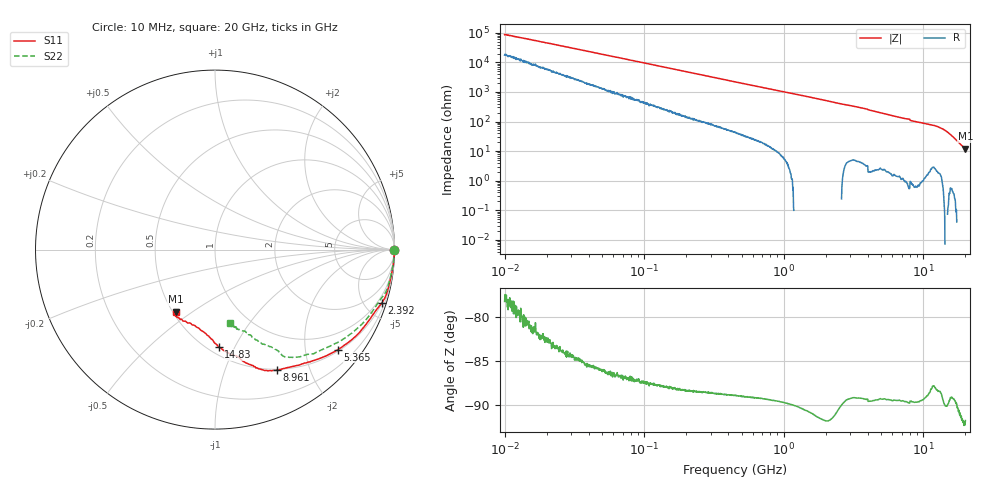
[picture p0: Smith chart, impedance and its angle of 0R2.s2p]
!Keysight Technologies,P5008B,MY61100088,A.16.20.02
!Date: Monday, October 30, 2023 15:49:30
!Correction: S11(C  2-Port  )
!S21(C  2-Port  )
!S12(C  2-Port  )
!S22(C  2-Port  )
!S2P File: Measurements: S11, S21, S12, S22:Log Frequency Sweep
# Hz S  dB  R 50
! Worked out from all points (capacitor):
!   1601 points, 10 MHz to 20 GHz, reference 50 ohm
!   read as one part in series: C = 181 fF near 10.39 MHz
!   lowest |Z| = 11.9 ohm at 20 GHz (marker M1)
!   S11 on the Smith chart (normalised r, x): 10 MHz: open; 2.392 GHz: 0.52, -6.36; 5.365 GHz: 0.54, -2.72; 8.961 GHz: 0.49, -1.52; 14.83 GHz: 0.56, -0.87; 20 GHz: 0.52, -0.43
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1e7  0.00 -0.1  -58.83 78.2  -58.91 78.9  -0.00 -0.1
3.555162e7  -0.00 -0.3  -48.41 84.8  -48.41 84.9  -0.00 -0.2
1.263918e8  -0.01 -1.0  -37.66 86.8  -37.66 86.9  -0.01 -0.8
4.472136e8  -0.02 -3.4  -26.88 85.7  -26.88 85.7  -0.02 -2.9
9.518201e8  -0.05 -7.1  -20.56 83.0  -20.57 83.0  -0.06 -6.1
1.589917e9  -0.09 -11.6  -16.38 80.1  -16.39 80.1  -0.10 -10.0
2.39224e9  -0.22 -17.8  -12.85 74.3  -12.85 74.2  -0.24 -15.3
3.846973e9  -0.58 -27.5  -9.39 64.0  -9.40 64.0  -0.58 -23.2
4.170543e9  -0.68 -30.7  -8.51 61.3  -8.51 61.3  -0.69 -25.8
5.364623e9  -1.09 -39.2  -6.59 53.1  -6.59 53.1  -1.09 -33.2
5.652411e9  -1.20 -41.2  -6.21 51.2  -6.22 51.2  -1.20 -35.0
7.697294e9  -1.92 -52.5  -4.49 40.6  -4.50 40.6  -1.90 -45.5
8.344716e9  -2.29 -59.4  -3.89 34.8  -3.90 34.7  -2.28 -50.2
8.961046e9  -2.45 -63.0  -3.64 31.8  -3.65 31.8  -2.44 -52.5
1.073392e10  -3.00 -69.8  -3.10 25.4  -3.10 25.4  -2.95 -57.0
1.22029e10  -3.55 -73.7  -2.68 22.3  -2.68 22.3  -3.48 -57.9
1.361179e10  -4.42 -79.3  -1.97 18.3  -1.97 18.3  -4.32 -61.7
1.482695e10  -5.30 -87.8  -1.44 12.5  -1.44 12.5  -5.22 -66.0
1.661757e10  -7.00 -101.8  -1.05 2.8  -1.06 2.8  -6.62 -72.7
1.827386e10  -7.27 -117.1  -0.94 -5.1  -0.95 -5.1  -6.98 -75.4
1.90721e10  -7.37 -121.3  -0.90 -7.7  -0.91 -7.7  -7.15 -77.0
2e10  -7.75 -122.2  -0.79 -9.4  -0.79 -9.4  -7.58 -78.4
